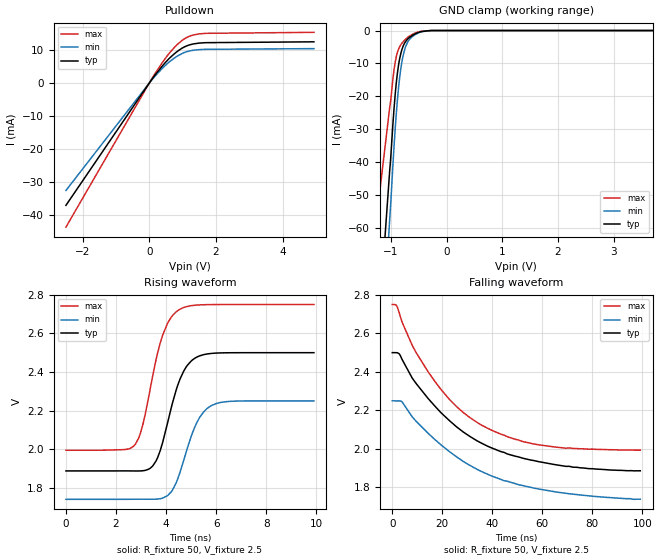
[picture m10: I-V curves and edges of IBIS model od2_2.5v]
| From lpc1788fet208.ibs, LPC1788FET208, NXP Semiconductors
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[Model]   od2_2.5v
Model_type I/O_open_drain
Vinl=7.500E-01
Vinh=1.750E+00
Vref=2.500E+00
Rref=2.000E+03
Cref=0.000E+00
Vmeas=1.250E+00
C_comp   5.160E-13   4.910E-13   5.420E-13
[Voltage Range]   2.500E+00   2.250E+00   2.750E+00
[POWER Clamp Reference]   2.500E+00   2.250E+00   2.750E+00
[GND Clamp Reference]   0.000E+00   0.000E+00   0.000E+00
[Pullup Reference]   2.500E+00   2.250E+00   2.750E+00
[Pulldown Reference]   0.000E+00   0.000E+00   0.000E+00
[Temperature Range]   25   85   -40
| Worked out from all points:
|   slope of the pulldown table from 0 to 0.375 V, typ, clamps not added: 75.7 ohm
|   GND clamp passes 1 mA (typ) near -0.56 V on its own axis
|   rising waveform, R_fixture 50, V_fixture 2.5: 20-80 % time 802ps typ, 818ps min, 783ps max; typ from 1.89 V to 2.5 V
|   falling waveform, R_fixture 50, V_fixture 2.5: 20-80 % time 31.4ns typ, 34.3ns min, 27.2ns max; typ from 2.5 V to 1.89 V
[GND Clamp]
-2.5V     -395.3mA   -473.6mA   -235.3mA
-1.024V   -42.81mA   -57.72mA   -23.54mA
-964.1mV  -28.07mA   -40.56mA   -14.51mA
-924.2mV  -19.36mA   -29.86mA   -9.595mA
-884.3mV  -12.91mA   -21.05mA   -6.612mA
-824.5mV  -7.051mA   -11.72mA   -4.351mA
-784.6mV  -4.877mA   -7.833mA   -3.476mA
-744.7mV  -3.531mA   -5.27mA    -2.76mA
-684.9mV  -2.339mA   -3.083mA   -1.885mA
-585.1mV  -1.199mA   -1.466mA   -903.2uA
-266mV    0A         0A         0A
5V        0A         0A         0A
[Pulldown]
-2.5V     -37.02mA   -32.52mA   -43.62mA
152.9mV   2.149mA    1.866mA    2.564mA
591.7mV   7.38mA     6.328mA    8.925mA
771.2mV   9.017mA    7.692mA    10.96mA
970.7mV   10.47mA    8.879mA    12.79mA
1.27V     11.72mA    9.839mA    14.4mA
1.629V    12.19mA    10.19mA    15.01mA
4.94V     12.49mA    10.42mA    15.36mA
[Rising Waveform]
R_fixture = 50
V_fixture = 2.5
V_fixture_min = 2.25
V_fixture_max = 2.75
0s        1.887V     1.739V     1.994V
2.376ns   1.887V     1.739V     1.998V
2.772ns   1.886V     1.74V      2.025V
3.069ns   1.887V     1.74V      2.126V
3.6ns     1.939V     1.74V      2.465V
4.059ns   2.137V     1.758V     2.653V
4.555ns   2.363V     1.879V     2.726V
5.148ns   2.471V     2.116V     2.746V
5.8ns     2.496V     2.225V     2.75V
9.901ns   2.5V       2.25V      2.75V
[Falling Waveform]
R_fixture = 50
V_fixture = 2.5
V_fixture_min = 2.25
V_fixture_max = 2.75
0s        2.5V       2.25V      2.75V
1.798ns   2.5V       2.249V     2.743V
3.896ns   2.465V     2.245V     2.66V
8.591ns   2.357V     2.157V     2.523V
17.28ns   2.219V     2.046V     2.346V
25.77ns   2.114V     1.958V     2.219V
35.07ns   2.034V     1.887V     2.128V
46.15ns   1.973V     1.832V     2.063V
58.04ns   1.935V     1.793V     2.022V
99.2ns    1.887V     1.739V     1.994V
[Ramp]
dV/dt_r   3.6807E-01/7.9470E-10   3.0650E-01/8.1600E-10   4.5371E-01/7.7670E-10
dV/dt_f   3.6807E-01/3.1494E-08   3.0650E-01/3.4327E-08   4.5371E-01/2.7399E-08
R_load = 50
